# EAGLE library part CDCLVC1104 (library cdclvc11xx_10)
CDCLVC1104 3.3V and 2.5V LVCMOS High-Performance Clock Buffer - 1:4 Fan-out Source: http://www.ti.com/lit/ds/symlink/cdclvc1104.pdf
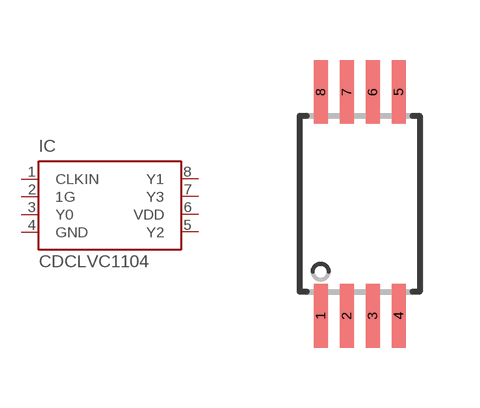
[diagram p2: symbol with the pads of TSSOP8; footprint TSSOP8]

Designator prefix IC

## CDCLVC1104PW (MF: Texas Instruments; MPN: CDCLVC1104; OC_FARNELL: 1829681; OC_NEWARK: 79R7910)  [TSSOP8]
1  CLKIN  in
2  1G  in
3  Y0  out
4  GND  pwr
5  Y2  out
6  VDD  pwr
7  Y3  out
8  Y1  out

## Footprint TSSOP8 (pad centres in mm)
TSSOP-8 Plastic Thin Srink Small Outline (PW) Source: http://www.ti.com/lit/ds/symlink/cdclvc1102.pdf
smd 0.35 x 1.6: 1 -0.975,-2.8; 2 -0.325,-2.8; 3 0.325,-2.8; 4 0.975,-2.8; 5 0.975,2.8; 6 0.325,2.8; 7 -0.325,2.8; 8 -0.975,2.8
